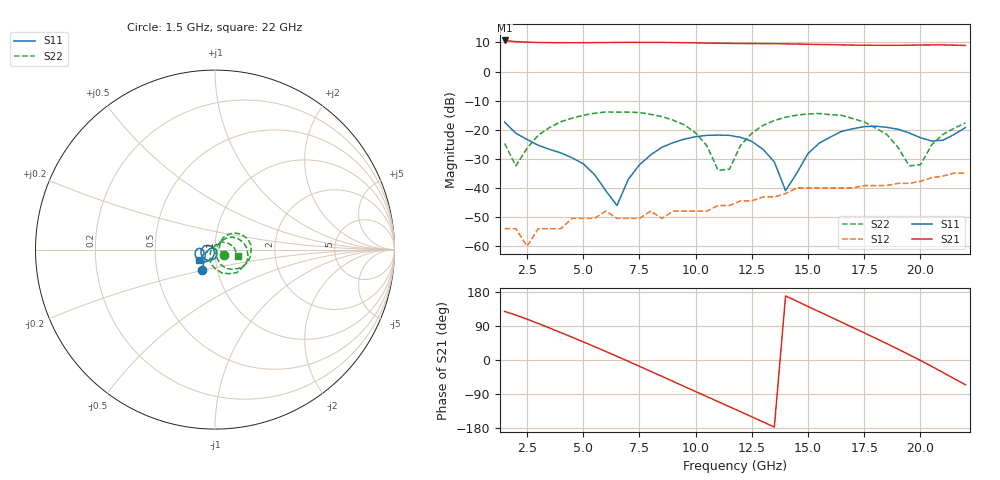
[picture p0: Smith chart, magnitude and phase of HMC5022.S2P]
! HMMC-5022
! Typical S-Parameters Ta=25 C, VDD=7V, ID=150mA or IDSS (whichever is less)
# ghz s ma r 50
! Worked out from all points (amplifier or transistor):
!   42 points, 1.5 GHz to 22 GHz, reference 50 ohm
!   highest |S21| = 10.7 dB at 1.5 GHz (marker M1)
!   |S21| within 3 dB of that: start of sweep to end of sweep
!   unconditionally stable (mu >= 1): start of sweep to end of sweep
!   at 5 GHz: K = 51.63, MAG = 10.0 dB, |S12| = -50.5 dB
!   at 12 GHz: K = 27.30, MAG = 9.7 dB, |S12| = -44.4 dB
!   at 22 GHz: K = 9.62, MAG = 9.1 dB, |S12| = -34.9 dB
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1.5  0.135 -121.1  3.416 128.2  0.002 179.5  0.058 -34.3
2  0.087 -134.8  3.255 118.6  0.002 154.9  0.024 14.4
2.5  0.068 -144.8  3.198 107.7  0.001 112.0  0.048 52.7
3.5  0.046 -162.1  3.135 84.4  0.002 93.3  0.109 49.0
5  0.026 163.8  3.125 47.8  0.003 57.4  0.177 26.0
6.5  0.005 20.1  3.161 9.6  0.003 15.3  0.201 -1.4
7  0.014 -41.8  3.171 -3.4  0.003 -7.8  0.201 -10.0
8.5  0.05 -91.7  3.161 -43.2  0.003 -34.8  0.168 -38.7
10  0.076 -131.8  3.105 -83.3  0.004 -64.3  0.088 -69.3
11  0.081 -158.6  3.06 -109.9  0.005 -78.0  0.02 -74.4
11.5  0.08 -170.8  3.042 -123.2  0.005 -91.6  0.021 57.4
12  0.074 176.3  3.028 -136.5  0.006 -102.3  0.054 55.4
13.5  0.028 136.3  3.003 -177.1  0.007 -133.0  0.144 24.5
14  0.009 150.7  2.984 169.0  0.008 -151.8  0.164 13.4
15.5  0.059 -110.5  2.914 127.4  0.01 174.1  0.19 -21.4
17  0.104 -143.1  2.841 85.6  0.01 130.4  0.155 -60.0
18  0.115 -164.9  2.828 57.5  0.011 103.1  0.107 -88.7
19  0.102 178.6  2.824 28.9  0.012 82.5  0.05 -124.8
19.5  0.088 175.2  2.836 14.0  0.012 70.6  0.024 -166.7
20.5  0.064 -174.9  2.868 -16.8  0.015 41.3  0.055 52.8
21  0.066 -159.7  2.869 -32.8  0.016 27.5  0.083 24.5
22  0.109 -146.8  2.811 -65.3  0.018 -1.8  0.131 -15.9
